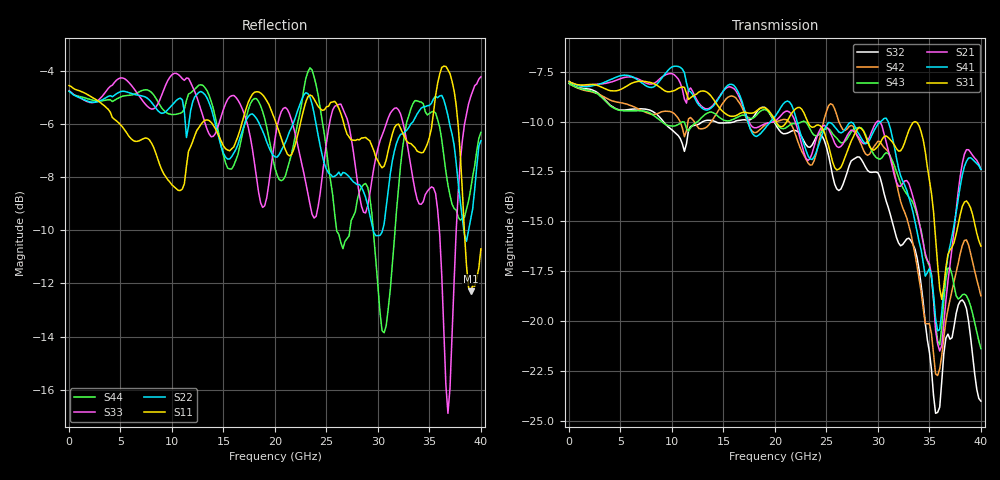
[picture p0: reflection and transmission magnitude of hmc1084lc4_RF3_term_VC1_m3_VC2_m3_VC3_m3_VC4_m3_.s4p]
!Agilent Technologies,N5224A,MY51441122,A.09.40.06
!Agilent N5224A: A.09.40.06
!Date: Thursday, June 19, 2014 00:52:33
!Correction: S11(Full 4 Port(1,2,3,4))
!S12(Full 4 Port(1,2,3,4))
!S13(Full 4 Port(1,2,3,4))
!S14(Full 4 Port(1,2,3,4))
!S21(Full 4 Port(1,2,3,4))
!S22(Full 4 Port(1,2,3,4))
!S23(Full 4 Port(1,2,3,4))
!S24(Full 4 Port(1,2,3,4))
!S31(Full 4 Port(1,2,3,4))
!S32(Full 4 Port(1,2,3,4))
!S33(Full 4 Port(1,2,3,4))
!S34(Full 4 Port(1,2,3,4))
!S41(Full 4 Port(1,2,3,4))
!S42(Full 4 Port(1,2,3,4))
!S43(Full 4 Port(1,2,3,4))
!S44(Full 4 Port(1,2,3,4))
!S4P File: Measurements: <S11,S12,S13,S14>,
!<S21,S22,S23,S24>,
!<S31,S32,S33,S34>,
!<S41,S42,S43,S44>:
# Hz S  dB  R 50
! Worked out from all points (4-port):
!   201 points, 10 MHz to 40 GHz, reference 50 ohm
!   strongest paths, dB at 10 MHz, 10.01 GHz, 20 GHz, 30 GHz, 40 GHz:
!     S31: -8.0, -8.5, -9.9, -11.2, -16.2
!     S41: -8.0, -7.3, -9.7, -10.1, -12.4
!     S21: -8.0, -7.6, -10.0, -10.0, -12.4
!     S43: -8.1, -10.2, -10.0, -11.9, -21.4
!     S42: -8.1, -9.5, -10.0, -11.0, -18.7
!     S32: -8.1, -10.4, -10.1, -12.6, -24.0
!   lowest |S11| = -12.3 dB at 39 GHz (marker M1), VSWR 1.64, Z = 30.6 + j2.84 ohm
!   |S11| at or under -10 dB: 38.39 GHz to end of sweep
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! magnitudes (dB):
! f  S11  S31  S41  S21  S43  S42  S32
! 10 MHz  -4.6  -8.0  -8.0  -8.0  -8.1  -8.1  -8.1
! 30.6 GHz  -7.6  -10.8  -9.8  -10.6  -11.7  -11.3  -13.6
! 31.8 GHz  -6.0  -11.4  -11.8  -13.0  -12.5  -13.1  -15.8
! 35.6 GHz  -4.9  -15.8  -19.9  -20.5  -20.2  -22.7  -24.6
! 36.8 GHz  -4.0  -16.7  -16.7  -18.0  -17.3  -19.4  -20.7
! 39 GHz  -12.3  -14.3  -11.8  -11.5  -19.3  -16.6  -20.8
! 40 GHz  -10.7  -16.2  -12.4  -12.4  -21.4  -18.7  -24.0
